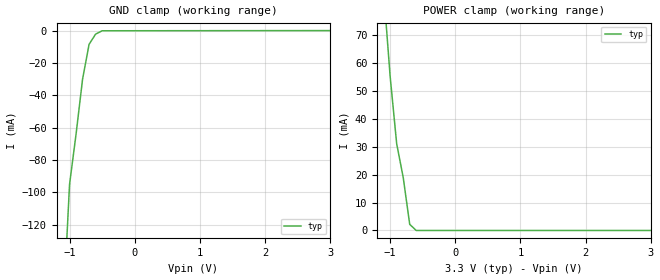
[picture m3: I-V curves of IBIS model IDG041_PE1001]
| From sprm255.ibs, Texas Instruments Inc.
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[Model]   IDG041_PE1001
Model_type   Input
Polarity   Non-Inverting
| signals   A, Y
Vinl = 0.8V
Vinh = 2.0V
|   typ   min   max
C_comp   3.8731p   3.7902p   4.0845p
|   typ   min   max
[Temperature Range]   25.0   -40   125
|   typ   min   max
[Voltage Range]   3.3V   3.0V   3.6V
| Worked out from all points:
|   GND clamp passes 1 mA (typ) near -0.54 V on its own axis
|   POWER clamp passes 1 mA (typ) near -0.65 V on its own axis
[GND_clamp]
|   Voltage   I(typ)   I(min)   I(max)
-3V       -1.8A      NA         NA
-2V       -900mA     NA         NA
-1V       -95mA      NA         NA
-900mV    -64mA      NA         NA
-800mV    -30mA      NA         NA
-700mV    -8.5mA     NA         NA
-600mV    -2.2mA     NA         NA
-500mV    -120uA     NA         NA
3V        0A         NA         NA
[POWER_clamp]
|   Voltage   I(typ)   I(min)   I(max)
-3V       900mA      NA         NA
-2V       360mA      NA         NA
-1V       55mA       NA         NA
-900mV    31mA       NA         NA
-800mV    19mA       NA         NA
-700mV    2.2mA      NA         NA
-600mV    0A         NA         NA
-500mV    0A         NA         NA
3V        0A         NA         NA
